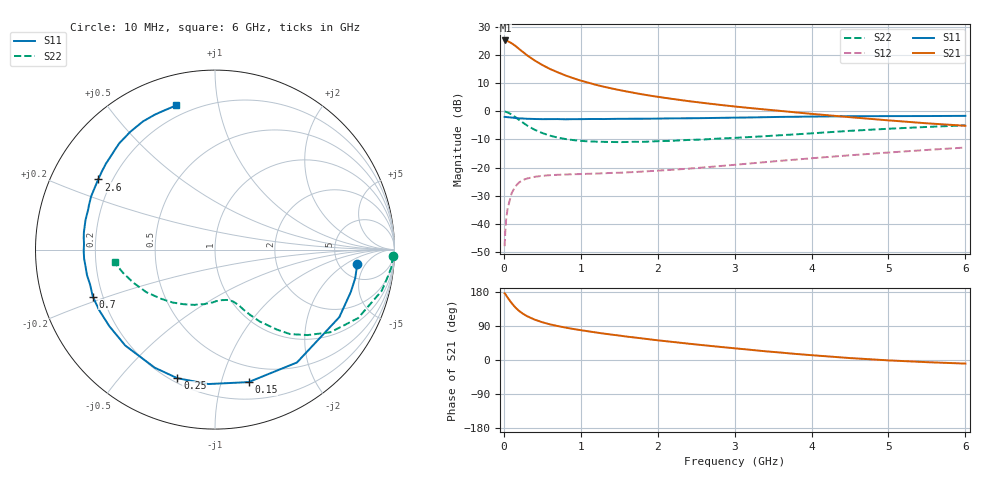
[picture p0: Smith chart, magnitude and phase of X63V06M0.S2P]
! SIEMENS Small Signal Semiconductors
! BFP193W
! Si NPN RF Bipolar Junction Transistor in SOT343
! VCE = 3 V  IC = 6 mA
! Common Emitter S-Parameters:  April 1994
# GHz  S  MA  R  50
!  f  S11  S21  S12  S22
! GHz  MAG  ANG  MAG  ANG  MAG  ANG  MAG  ANG
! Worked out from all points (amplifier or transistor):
!   40 points, 10 MHz to 6 GHz, reference 50 ohm
!   highest |S21| = 25.2 dB at 20 MHz (marker M1)
!   |S21| within 3 dB of that: start of sweep to 197 MHz
!   unconditionally stable (mu >= 1): 1.571 GHz to 4.28 GHz
!   at 200 MHz: K = 0.16, MSG = 23.7 dB, |S12| = -25.3 dB
!   at 1.5 GHz: K = 0.97, MSG = 14.7 dB, |S12| = -21.8 dB
!   at 6 GHz: K = 0.92, MSG = 3.9 dB, |S12| = -12.9 dB
!   lowest NFmin = 1.20 dB at 450 MHz
!   S11 on the Smith chart (normalised r, x): 10 MHz: 7.43, -3.23; 150 MHz: 0.35, -1.22; 250 MHz: 0.22, -0.73; 700 MHz: 0.16, -0.18; 2.6 GHz: 0.15, +0.27; 6 GHz: 0.14, +0.76
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0.01  0.7971 -5.7  18.19 175.9  0.004 87.4  0.9924 -2.0
0.02  0.7972 -11.6  18.26 173.7  0.0077 84.1  0.9871 -5.8
0.05  0.7883 -28.5  17.77 164.4  0.019 76.2  0.9568 -13.9
0.1  0.7772 -54.0  16.32 150.5  0.0347 63.6  0.8838 -25.6
0.15  0.7616 -75.8  14.62 138.5  0.0464 53.9  0.7907 -35.6
0.2  0.7499 -92.8  12.82 129.2  0.0545 46.5  0.7023 -42.7
0.25  0.7467 -106.3  11.33 121.9  0.0601 40.8  0.6292 -48.4
0.3  0.7386 -117.1  9.993 115.8  0.0638 36.7  0.5628 -52.3
0.4  0.7319 -133.1  8.052 106.6  0.0685 30.9  0.4717 -58.1
0.5  0.7271 -144.1  6.68 99.6  0.0714 27.7  0.4118 -61.8
0.6  0.7283 -152.3  5.68 94.1  0.0732 25.7  0.3701 -64.6
0.7  0.7295 -159.0  4.96 89.6  0.0744 24.8  0.3415 -66.5
0.9  0.7272 -168.7  3.903 82.0  0.0762 24.0  0.3086 -70.4
1.1  0.731 -176.1  3.232 75.6  0.0776 24.7  0.2921 -74.1
1.3  0.7305 177.6  2.746 69.7  0.0792 26.1  0.2867 -78.1
1.6  0.7378 169.6  2.255 61.7  0.0822 28.9  0.2853 -84.0
2.2  0.7511 156.8  1.659 47.6  0.0915 34.8  0.3002 -97.1
2.6  0.7591 149.0  1.409 38.9  0.1006 38.4  0.3164 -106.1
3.2  0.7789 138.4  1.147 27.0  0.1183 41.4  0.3497 -119.4
4.5  0.8193 119.3  0.788 5.1  0.1655 41.3  0.4506 -148.3
5.5  0.8255 109.7  0.613 -5.7  0.2059 37.4  0.5286 -165.8
6  0.8318 105.1  0.554 -9.5  0.2275 35.1  0.5637 -172.7
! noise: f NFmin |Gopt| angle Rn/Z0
0.45  1.2  0.25  114  0.13
0.9  1.25  0.37  150  0.12
1.8  2  0.55  -158  0.12
